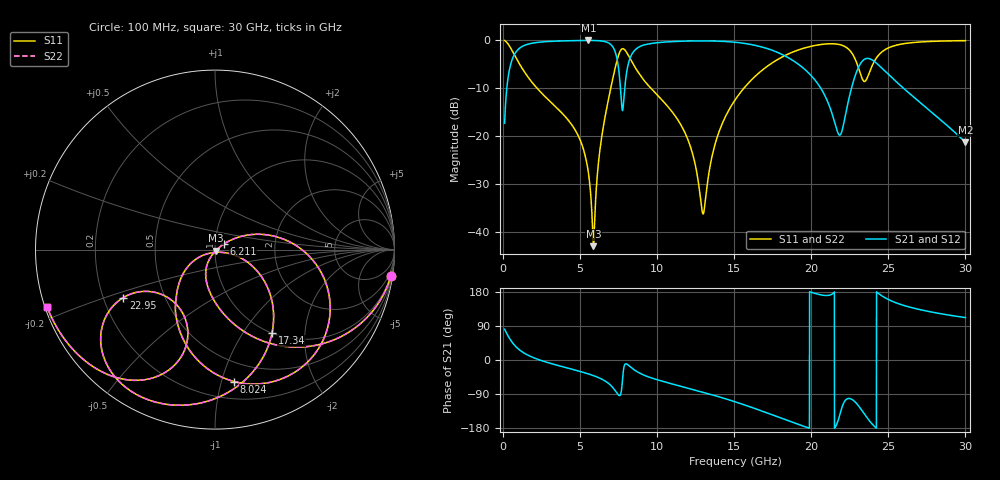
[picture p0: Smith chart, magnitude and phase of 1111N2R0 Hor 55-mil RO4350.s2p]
# GHz S MA R 50
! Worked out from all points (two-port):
!   3201 points, 100 MHz to 30 GHz, reference 50 ohm
!   highest |S21| = -0.06 dB at 5.538 GHz (marker M1); lowest = -21.3 dB at 30 GHz (marker M2)
!   |S21| within 3 dB of the highest: 722.4 MHz to 7.334 GHz (6.611 GHz wide, 164 % of centre); 8.336 GHz to 18.16 GHz (9.821 GHz wide, 74.1 % of centre)
!   lowest |S11| = -42.9 dB at 5.865 GHz (marker M3), VSWR 1.01, Z = 50.5 - j0.541 ohm
!   |S11| at or under -10 dB: 2.202 GHz to 6.988 GHz (4.786 GHz wide, 104 % of centre); 9.588 GHz to 15.63 GHz (6.041 GHz wide, 47.9 % of centre)
!   |S22| runs from -42.9 to -0.1 dB; largest |S21 - S12| = 0
!   S11 on the Smith chart (normalised r, x): 100 MHz: 1, -13; 6.211 GHz: 1.10, +0.07; 8.024 GHz: 0.33, -1.10; 17.34 GHz: 1.00, -1.36; 22.95 GHz: 0.28, -0.23; 30 GHz: 0.01, -0.17
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0.1  0.9906 -8.6  0.1361 81.4  0.1361 81.4  0.9906 -8.6
0.585875  0.7791 -43.0  0.6262 46.9  0.6262 46.9  0.7791 -43.0
1.632375  0.4098 -77.4  0.9108 12.4  0.9108 12.4  0.4098 -77.4
5.089563  0.08387 -118.7  0.9922 -31.2  0.9922 -31.2  0.08387 -118.7
5.538062  0.04141 -119.5  0.9934 -36.7  0.9934 -36.7  0.04141 -119.5
5.865094  0.007137 -48.6  0.9923 -41.2  0.9923 -41.2  0.007137 -48.6
6.210813  0.05691 32.3  0.987 -46.8  0.987 -46.8  0.05691 32.3
7.070437  0.3655 10.5  0.8737 -70.4  0.8737 -70.4  0.3655 10.5
7.50025  0.7026 -24.3  0.4987 -92.9  0.4987 -92.9  0.7026 -24.3
7.752531  0.8148 -54.3  0.1846 -50.6  0.1846 -50.6  0.8148 -54.3
8.0235  0.7431 -81.7  0.4687 -10.7  0.4687 -10.7  0.7431 -81.7
10.06978  0.262 -138.3  0.9433 -52.9  0.9433 -52.9  0.262 -138.3
11.97591  0.09353 -154.6  0.9791 -74.0  0.9791 -74.0  0.09353 -154.6
12.97569  0.01547 -85.7  0.9832 -85.1  0.9832 -85.1  0.01547 -85.7
15.05  0.2378 -24.7  0.9514 -110.3  0.9514 -110.3  0.2378 -24.7
17.33922  0.5624 -55.6  0.7979 -142.8  0.7979 -142.8  0.5624 -55.6
20.03956  0.8674 -97.3  0.4191 178.1  0.4191 178.1  0.8674 -97.3
21.84291  0.8994 -128.9  0.1024 -145.6  0.1024 -145.6  0.8994 -128.9
22.95481  0.576 -152.4  0.4752 -115.5  0.4752 -115.5  0.576 -152.4
23.79575  0.4719 -108.8  0.6396 -161.8  0.6396 -161.8  0.4719 -108.8
25.01978  0.8336 -119.3  0.4378 159.2  0.4378 159.2  0.8336 -119.3
30  0.9888 -161.1  0.08623 112.0  0.08623 112.0  0.9888 -161.1
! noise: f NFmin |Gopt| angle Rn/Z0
0.1  0.001809  0.908  2.998  0.004316
3.417  0.0114  0.539  26.84  0.004168
6.743  0.05673  0.7932  46.76  0.04785
10.06  0.06104  0.7335  68.77  0.03148
13.39  0.05939  0.6615  87.17  0.01827
16.7  0.08614  0.7105  103.4  0.02354
20.03  0.2432  0.8697  120.8  0.09949
23.35  0.465  0.9179  137.6  0.1661
26.67  0.3347  0.881  150.4  0.04209
30  0.5896  0.9335  164.1  0.04007
